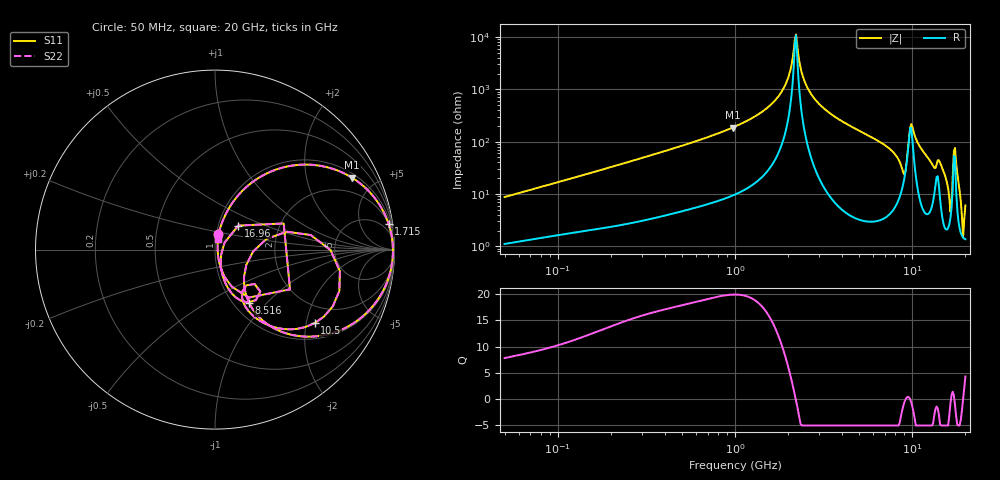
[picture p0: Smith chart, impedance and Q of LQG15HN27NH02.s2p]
!Murata Part Number: LQG15HN27NH02
!These Parameters are Measured in Series Mode Connection
!  o--[Z]--o
!Port1  Port2
!  o-------o
!Freq. Start=50[MHz] Stop=20[GHz], 401[Steps]
# Hz S RI R 50
!Freq.(Hz) S11(Real) S11(Imag) S21(Real) S21(Imag) S12(Real) S12(Imag) S22(Real) S22(Imag)
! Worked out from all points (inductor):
!   401 points, 50 MHz to 20 GHz, reference 50 ohm
!   read as one part in series: L = 27.2 nH near 51.52 MHz
!   highest Q = 19.9 at 970.5 MHz (marker M1), where L = 30.4 nH
!   self-resonance near 2.179 GHz
!   S11 on the Smith chart (normalised r, x): 50 MHz: 1.02, +0.17; 1.715 GHz: 2, +13; 8.516 GHz: 1.18, -0.80; 10.5 GHz: 1.43, -2.24; 16.96 GHz: 1.24, +0.34; 20 GHz: 1.03, +0.12
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5e7  0.0182 0.0842  0.9818 -0.0842  0.9818 -0.0842  0.0182 0.0842
1.364002e8  0.0643 0.2065  0.9357 -0.2065  0.9357 -0.2065  0.0643 0.2065
3.721004e8  0.2826 0.4214  0.7174 -0.4214  0.7174 -0.4214  0.2826 0.4214
9.70487e8  0.7642 0.4001  0.2358 -0.4001  0.2358 -0.4001  0.7642 0.4001
1e9  0.7789 0.3906  0.2211 -0.3906  0.2211 -0.3906  0.7789 0.3906
1.714689e9  0.9667 0.1448  0.0333 -0.1448  0.0333 -0.1448  0.9667 0.1448
1.962148e9  0.9855 0.0681  0.0145 -0.0681  0.0145 -0.0681  0.9855 0.0681
2.211938e9  0.9914 -0.00244  0.00856 0.00244  0.00856 0.00244  0.9914 -0.00244
2.419936e9  0.9889 -0.0561  0.0111 0.0561  0.0111 0.0561  0.9889 -0.0561
2.728004e9  0.9759 -0.1278  0.0241 0.1278  0.0241 0.1278  0.9759 -0.1278
7.442007e9  0.3589 -0.4529  0.6411 0.4529  0.6411 0.4529  0.3589 -0.4529
8.516016e9  0.1897 -0.2965  0.8103 0.2965  0.8103 0.2965  0.1897 -0.2965
9.041845e9  0.1743 -0.0855  0.8257 0.0855  0.8257 0.0855  0.1743 -0.0855
9.457416e9  0.4004 0.0997  0.5996 -0.0997  0.5996 -0.0997  0.4004 0.0997
9.892087e9  0.6958 -0.1199  0.3042 0.1199  0.3042 0.1199  0.6958 -0.1199
1.050288e10  0.5546 -0.4098  0.4454 0.4098  0.4454 0.4098  0.5546 -0.4098
1.460232e10  0.1415 -0.2834  0.8585 0.2834  0.8585 0.2834  0.1415 -0.2834
1.621653e10  0.0318 -0.0784  0.9682 0.0784  0.9682 0.0784  0.0318 -0.0784
1.696185e10  0.1296 0.1337  0.8704 -0.1337  0.8704 -0.1337  0.1296 0.1337
1.774144e10  0.1883 -0.2674  0.8117 0.2674  0.8117 0.2674  0.1883 -0.2674
1.912117e10  0.0168 -0.0334  0.9832 0.0334  0.9832 0.0334  0.0168 -0.0334
2e10  0.0168 0.0571  0.9832 -0.0571  0.9832 -0.0571  0.0168 0.0571
